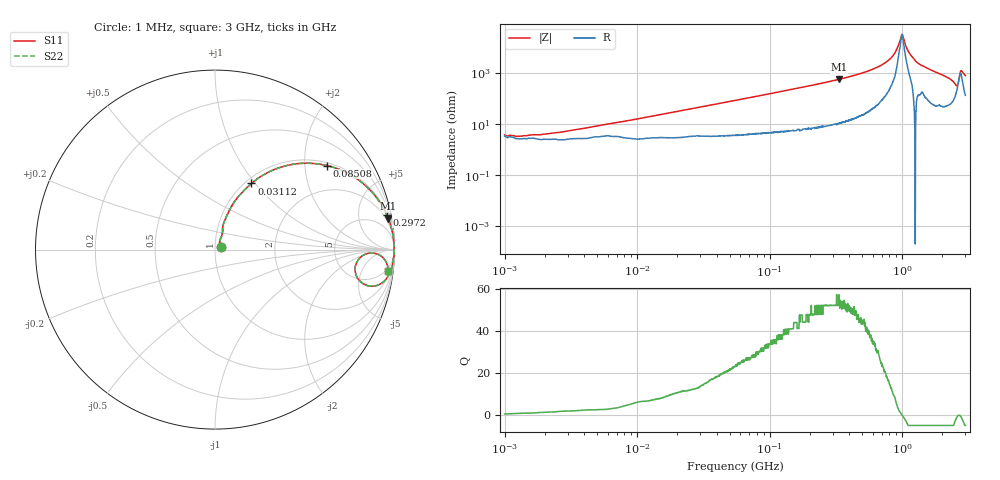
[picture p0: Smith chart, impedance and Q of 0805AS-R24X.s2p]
!s-Parameter Generated by FASTRON Sdn. Bhd.
!FASTRON P/N : 0805AS-R24X
!Keysight Technologies: E4991B_MY54100416_A.01.15
!Date: Mon Jun 15 12:53:14 2026
!Version  :Rev01  Mon Jun 15 12:53:14 2026
!Data & Calibration Information:
!Freq  S11  S21  S12  S22
!PortZ  Port1:50+j0  Port2:50+j0
!When reading reference impedance value at option line is always used.
! Remarks : This data is being provided solely for informational purposes.
# Hz S dB R 50
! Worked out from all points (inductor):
!   1601 points, 1 MHz to 3 GHz, reference 50 ohm
!   read as one part in series: L = 248 nH near 6.369 MHz
!   highest Q = 52.6 at 333.5 MHz (marker M1), where L = 269 nH
!   self-resonance near 997.7 MHz
!   S11 on the Smith chart (normalised r, x): 1 MHz: 1.07, +0.03; 31.12 MHz: 1.07, +0.96; 85.08 MHz: 1.09, +2.59; 297.2 MHz: 1.19, +9.79; 3 GHz: 4, -16
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1000000  -28.80 23.9  -0.29 -0.9  -0.29 -0.9  -28.80 23.9
1869176  -28.50 48.3  -0.21 -1.6  -0.21 -1.6  -28.50 48.3
3804036  -23.90 62.4  -0.24 -3.3  -0.24 -3.3  -23.90 62.4
1.447069e7  -13.40 70.3  -0.45 -12.3  -0.45 -12.3  -13.40 70.3
3.111637e7  -7.52 61.2  -1.13 -24.8  -1.13 -24.8  -7.52 61.2
5.504702e7  -4.01 48.5  -2.50 -39.0  -2.50 -39.0  -4.01 48.5
8.507507e7  -2.16 36.9  -4.43 -51.2  -4.43 -51.2  -2.16 36.9
2.083556e8  -0.44 16.9  -10.70 -71.9  -10.70 -71.9  -0.44 16.9
2.972367e8  -0.21 11.5  -14.00 -77.4  -14.00 -77.4  -0.21 11.5
3.334925e8  -0.16 10.1  -15.20 -78.9  -15.20 -78.9  -0.16 10.1
5.753936e8  -0.04 4.5  -22.20 -84.0  -22.20 -84.0  -0.04 4.5
7.925923e8  -0.02 1.8  -30.10 -84.6  -30.10 -84.6  -0.02 1.8
8.760197e8  -0.02 1.0  -35.20 -82.4  -35.20 -82.4  -0.02 1.0
9.730857e8  -0.03 0.2  -46.80 -46.2  -46.80 -46.2  -0.03 0.2
1.002744e9  -0.03 -0.0  -50.00 11.2  -50.00 11.2  -0.03 -0.0
1.142072e9  -0.02 -1.0  -35.00 81.7  -35.00 81.7  -0.02 -1.0
1.353887e9  -0.03 -2.6  -26.80 83.8  -26.80 83.8  -0.03 -2.6
2.210833e9  -0.21 -8.6  -16.50 76.7  -16.50 76.7  -0.21 -8.6
2.51802e9  -1.03 -13.2  -12.20 56.3  -12.20 56.3  -1.03 -13.2
2.607784e9  -2.05 -8.7  -12.00 28.6  -12.00 28.6  -2.05 -8.7
2.797026e9  -0.47 -3.4  -22.20 46.0  -22.20 46.0  -0.47 -3.4
3e9  -0.25 -7.0  -18.20 73.4  -18.20 73.4  -0.25 -7.0
